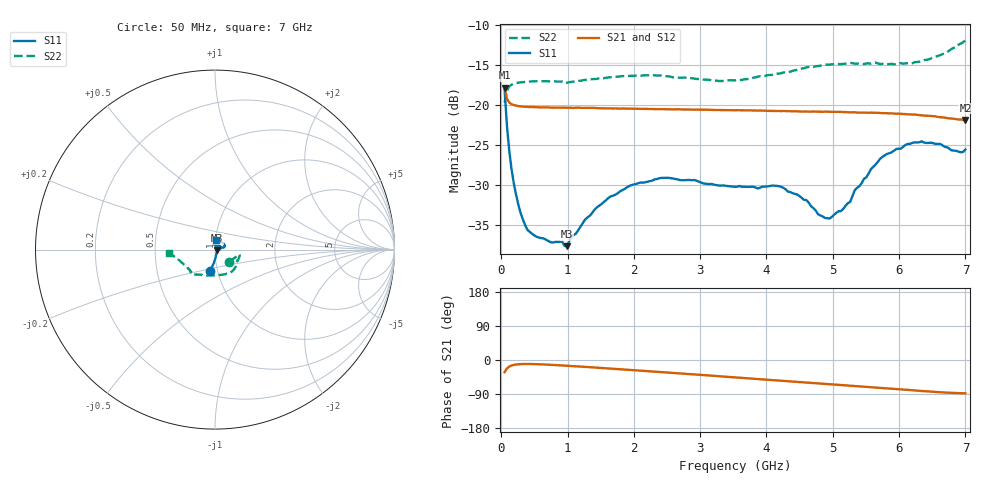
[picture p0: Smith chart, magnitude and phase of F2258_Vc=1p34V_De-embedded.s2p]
! Integrated Device Technology
! Corporate Headquarters
! 6024 Silver Creek Valley Road
! San Jose, CA 95138  USA
! Phone:  1-408-284-8200
! Toll Free:  1-800-223-1366
! Webpage:  http://www.idt.com/
! Timing and RF Division
! 515 Groton Road, Suite 102
! Westford, MA 01886-6024
! Device:  F2258
! Description: Voltage Variable RF Attenuator
! Frequency:  50.0 -  6000.00 MHz
! Package:  3x3 mm Thin QFN Plastic Package: 16 pin
! Ports:  2 RF, 2 DC
!  Pin  1  = NC
!  Pin  2  = NC
!  Pin  3  = RF2  = Port 2
!  Pin  4  = GND
!  Pin  5  = Vdd
!  Pin  6  = NC
!  Pin  7  = VCTRL
!  Pin  8  = NC
!  Pin  9  = GND
!  Pin 10  = RF1  = Port 1
!  Pin 11  = NC
!  Pin 12  = NC
!  Pin 13  = NC
!  Pin 14  = NC
!  Pin 15  = NC
!  Pin 16  = NC
! Vcntrl:  1.340 Volts
! Vdd:  +3.300 Volts
! Current:  1.167 mA
! Data:  The device was measured on a the F2258 evaluation board which has
!  individual transmission lines to the RF pins.  Data was collected
!  using a calibrated network analyzer.  The evaluation board was
!  de-embedded using a TRL calibration technique.
!  The reference plane is the edge of the package pin.
! Misc:  SN 10
!  Action Tracker AT0285
! Date Measured:  2014-12-10
! Date:  2016-01-13  MJV
! Note:
!  Integrated Device Technology supplies this data as a sample of measured
!  data at the package pin for this product.  Your particular data for this
!  product may vary.
!  Data was taken at 25 degrees C.
!  Integrated Device Technology reserves the right to change this data at anytime.
!Freq_(GHz)  S11M_(dB)  S11P_(deg)  S21M_(dB)  S21P_(deg)  S12M_(dB)  S12P_(deg)  S22M_(dB)  S22P_(deg)
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# GHz S dB R 50
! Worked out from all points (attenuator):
!   201 points, 50 MHz to 7 GHz, reference 50 ohm
!   highest |S21| = -17.79 dB at 50 MHz (marker M1); lowest = -21.8 dB at 7 GHz (marker M2)
!   lowest |S11| = -37.6 dB at 988.2 MHz (marker M3), VSWR 1.03, Z = 51.2 - j0.509 ohm
!   |S11| at or under -10 dB: start of sweep to end of sweep
!   |S22| runs from -19.6 to -11.9 dB; largest |S21 - S12| = 0.0004
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0.05  -18.05 -103.1  -17.79 -32.0  -17.79 -32.0  -19.63 -39.6
0.08475  -22.50 -94.9  -19.16 -22.4  -19.17 -22.4  -18.16 -19.2
0.15425  -27.99 -84.2  -19.84 -14.6  -19.84 -14.6  -17.40 -12.4
0.2585  -32.47 -70.3  -20.09 -11.2  -20.06 -11.2  -17.15 -11.2
0.36275  -35.05 -57.2  -20.16 -10.5  -20.15 -10.5  -17.06 -12.4
0.5365  -36.44 -39.5  -20.23 -11.0  -20.21 -11.0  -16.97 -15.5
0.98825  -37.61 -22.2  -20.29 -15.1  -20.29 -15.1  -17.16 -26.5
1.2315  -34.70 -8.1  -20.30 -17.7  -20.31 -17.7  -16.84 -31.8
1.6485  -31.38 1.8  -20.38 -22.7  -20.36 -22.7  -16.48 -40.7
2.37825  -29.12 21.2  -20.47 -31.5  -20.49 -31.5  -16.26 -56.1
3.525  -30.18 74.7  -20.61 -45.9  -20.61 -45.9  -16.87 -93.5
4.22  -30.18 99.8  -20.71 -54.7  -20.72 -54.7  -15.98 -117.6
4.7065  -32.84 86.9  -20.75 -60.8  -20.76 -60.8  -15.18 -127.2
4.94975  -34.14 61.5  -20.80 -63.8  -20.82 -63.8  -14.89 -130.2
5.1235  -33.21 42.8  -20.81 -66.0  -20.80 -66.0  -14.83 -132.1
5.2625  -32.06 28.4  -20.88 -67.7  -20.88 -67.7  -14.69 -133.5
5.332  -30.59 23.3  -20.86 -68.7  -20.88 -68.6  -14.79 -133.7
5.57525  -27.97 15.3  -20.91 -71.7  -20.92 -71.7  -14.78 -137.0
5.85325  -25.98 14.8  -20.99 -75.3  -20.99 -75.4  -14.82 -141.3
6.33975  -24.49 24.0  -21.23 -81.8  -21.23 -81.8  -14.46 -153.4
6.9305  -25.86 73.6  -21.75 -87.7  -21.75 -87.7  -12.26 -173.4
7  -25.51 83.8  -21.83 -87.9  -21.83 -88.0  -11.87 -176.0
